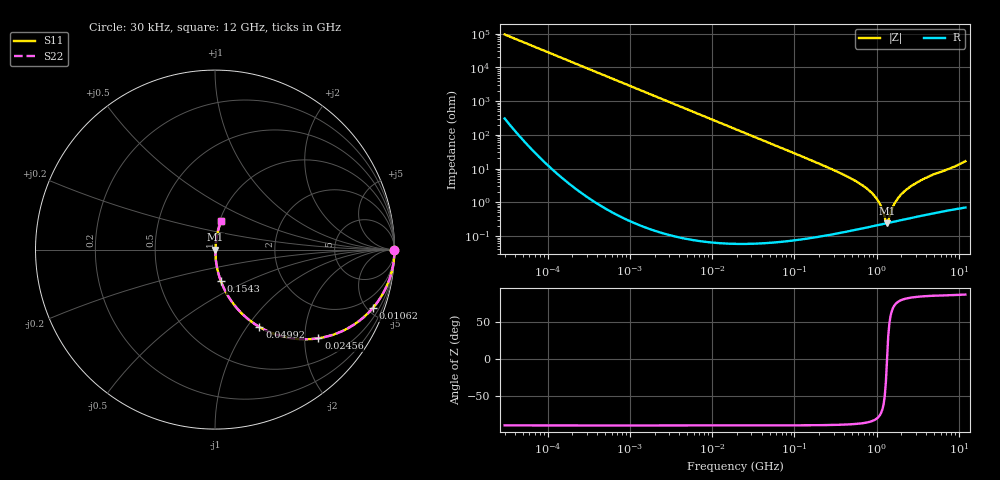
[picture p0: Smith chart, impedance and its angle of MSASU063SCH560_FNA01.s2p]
! MSASU063SCH560_FNA01  S-PARAMETER MODEL  ( General Type )
! Model Generated by TAIYO YUDEN Corporation (http://www.ty-top.com)
! Version 4.0
! TAIYO YUDEN Control No. 120810
! Copyright(c) 2002 TAIYO YUDEN CO.,LTD. All Rights Reserved.
! Product Description (link to TY-COMPAS)
! https://ds.yuden.co.jp/TYCOMPAS/or/detail?pn=MSASU063SCH560JFNA01&u=M
! Products Name : Multilayer Ceramic Capacitors
! Characteristics :
!  Capacitance : 56 pF , Rated Voltage : 50V , TCC : CH / C0H
!  Case Size : 0.6 x 0.3 / 0.024 x 0.012 [mm/inch] , Thickness : 0.3 / 0.012 [mm/inch]
!  (Conditions: Temperature = 25 degC , DC Bias Current/Voltage = 0A / 0V)
! External Node Assignments :
!  1  o---| |---o  2
! GND o---------o GND
! Frequency Range : 0.03MHz  -  12000MHz  [ 401 STEP ]
# MHz S RI R 50
! Freq[MHz].  S11 Real  S11 Imag  S21 Real  S21 Imag  S12 Real  S12 Imag  S22 Real  S22 Imag
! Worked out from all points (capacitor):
!   401 points, 30 kHz to 12 GHz, reference 50 ohm
!   read as one part in series: C = 55.6 pF near 32 kHz
!   lowest |Z| = 240 mohm at 1.339 GHz (marker M1)
!   series resonance near 1.34 GHz, so ESL is about 250 pH
!   S11 on the Smith chart (normalised r, x): 30 kHz: open; 10.62 MHz: 1.00, -5.39; 24.56 MHz: 1.00, -2.33; 49.92 MHz: 1.00, -1.14; 154.3 MHz: 1.00, -0.37; 12 GHz: 1.01, +0.33
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0.03  1 -0.00105  4.47e-06 0.00105  4.47e-06 0.00105  1 -0.00105
0.260295  0.9999 -0.0091  8.43e-05 0.0091  8.43e-05 0.0091  0.9999 -0.0091
2.258455  0.9938 -0.0784  0.0062 0.0784  0.0062 0.0784  0.9938 -0.0784
10.61839  0.8789 -0.3261  0.1211 0.3261  0.1211 0.3261  0.8789 -0.3261
18.97367  0.6945 -0.4604  0.3055 0.4604  0.3055 0.4604  0.6945 -0.4604
24.55797  0.5757 -0.494  0.4243 0.494  0.4243 0.494  0.5757 -0.494
49.92358  0.247 -0.4307  0.753 0.4307  0.753 0.4307  0.247 -0.4307
83.63502  0.1046 -0.305  0.8954 0.305  0.8954 0.305  0.1046 -0.305
154.3427  0.0332 -0.1767  0.9668 0.1767  0.9668 0.1767  0.0332 -0.1767
164.6252  0.0293 -0.166  0.9707 0.166  0.9707 0.166  0.0293 -0.166
433.1624  0.00482 -0.0588  0.9952 0.0588  0.9952 0.0588  0.00482 -0.0588
749.4426  0.00245 -0.0261  0.9975 0.0261  0.9975 0.0261  0.00245 -0.0261
1034.641  0.00221 -0.0111  0.9978 0.0111  0.9978 0.0111  0.00221 -0.0111
1139.739  0.00225 -0.0069  0.9978 0.0069  0.9978 0.0069  0.00225 -0.0069
1255.512  0.00232 -0.00276  0.9977 0.00276  0.9977 0.00276  0.00232 -0.00276
1339.156  0.0024 -1.85e-05  0.9976 1.85e-05  0.9976 1.85e-05  0.0024 -1.85e-05
1428.372  0.00249 0.00275  0.9975 -0.00275  0.9975 -0.00275  0.00249 0.00275
1573.464  0.00265 0.00677  0.9973 -0.00677  0.9973 -0.00677  0.00265 0.00677
1733.294  0.00286 0.0108  0.9971 -0.0108  0.9971 -0.0108  0.00286 0.0108
2471.32  0.00402 0.0267  0.996 -0.0267  0.996 -0.0267  0.00402 0.0267
4275.791  0.00763 0.0569  0.9924 -0.0569  0.9924 -0.0569  0.00763 0.0569
12000  0.0331 0.159  0.9669 -0.159  0.9669 -0.159  0.0331 0.159
